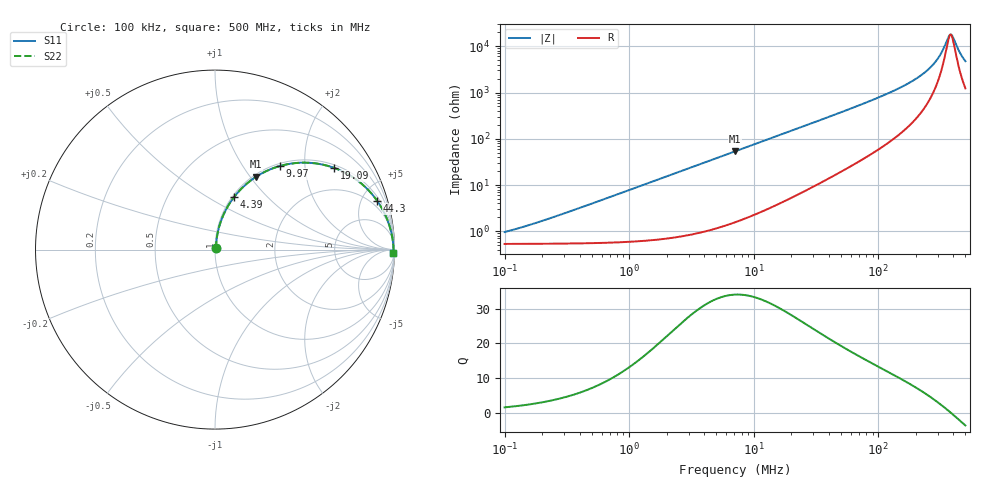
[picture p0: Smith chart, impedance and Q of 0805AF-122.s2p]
# MHz  S  MA  R  50
!Freq  MagS11  AngS11  MagS21  AngS21  MagS12  AngS12  MagS22  AngS22
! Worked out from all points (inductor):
!   801 points, 100 kHz to 500 MHz, reference 50 ohm
!   read as one part in series: L = 1.26 uH near 204.2 kHz
!   highest Q = 34.1 at 7.09 MHz (marker M1), where L = 1.2 uH
!   self-resonance near 377 MHz
!   S11 on the Smith chart (normalised r, x): 100 kHz: 1.01, +0.02; 4.39 MHz: 1.02, +0.67; 9.97 MHz: 1.04, +1.50; 19.09 MHz: 1.10, +2.84; 44.3 MHz: 1.32, +6.58; 500 MHz: 26, -92
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0.1  0.009584 55.9  0.9947 -0.5  0.9947 -0.5  0.009584 55.9
0.1758765  0.01491 68.2  0.9946 -0.8  0.9946 -0.8  0.01491 68.2
0.4168304  0.03303 78.6  0.994 -1.9  0.994 -1.9  0.03303 78.6
1.719065  0.1306 79.6  0.9849 -7.5  0.9849 -7.5  0.1306 79.6
4.389648  0.3135 69.9  0.9398 -18.3  0.9398 -18.3  0.3135 69.9
7.089654  0.466 60.6  0.8712 -27.8  0.8712 -27.8  0.466 60.6
9.969539  0.5909 52.1  0.7893 -36.2  0.7893 -36.2  0.5909 52.1
13.72372  0.705 43.4  0.6872 -44.8  0.6872 -44.8  0.705 43.4
19.09393  0.8049 34.5  0.566 -53.6  0.566 -53.6  0.8049 34.5
29.55184  0.8962 24.1  0.4085 -63.6  0.4085 -63.6  0.8962 24.1
44.29899  0.9441 16.6  0.2868 -70.6  0.2868 -70.6  0.9441 16.6
121.8757  0.9863 5.8  0.1007 -79.3  0.1007 -79.3  0.9863 5.8
188.6281  0.9914 3.2  0.05553 -79.5  0.05553 -79.5  0.9914 3.2
254.1851  0.9933 1.7  0.0308 -76.6  0.0308 -76.6  0.9933 1.7
304.6503  0.994 0.9  0.01738 -69.3  0.01738 -69.3  0.994 0.9
328.2371  0.9942 0.6  0.01226 -61.5  0.01226 -61.5  0.9942 0.6
361.2657  0.9944 0.2  0.00677 -34.0  0.00677 -34.0  0.9944 0.2
376.9927  0.9945 0.0  0.005592 -7.1  0.005592 -7.1  0.9945 0.0
385.1111  0.9945 -0.0  0.005594 8.8  0.005594 8.8  0.9945 -0.0
397.6177  0.9945 -0.2  0.006361 30.0  0.006361 30.0  0.9945 -0.2
451.8398  0.9945 -0.7  0.01373 66.0  0.01373 66.0  0.9945 -0.7
500  0.9944 -1.2  0.02094 73.8  0.02094 73.8  0.9944 -1.2
